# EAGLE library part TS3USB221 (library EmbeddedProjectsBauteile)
USB-Hub
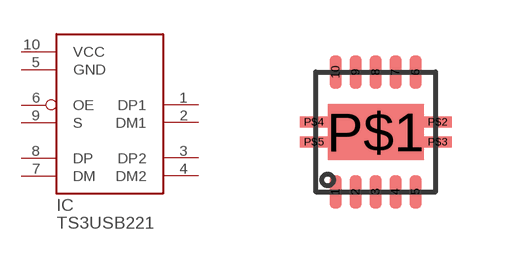
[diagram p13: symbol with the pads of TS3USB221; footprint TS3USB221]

Designator prefix IC

## TS3USB221 (EP: 400184)  [TS3USB221]
1  DP1
2  DM1
3  DP2
4  DM2
5  GND
6  OE
7  DM
8  DP
9  S
10  VCC  pwr

## Footprint TS3USB221 (pad centres in mm)
smd 0.3 x 0.85: 1 -1,-1.5; 2 -0.5,-1.5; 3 0,-1.5; 4 0.5,-1.5; 5 1,-1.5; 6 1,1.5; 7 0.5,1.5; 8 0,1.5; 9 -0.5,1.5; 10 -1,1.5
smd 2.4 x 1.4: P$1 0,0
smd 0.7 x 0.28: P$2 1.55,0.25; P$3 1.55,-0.25; P$4 -1.55,0.25; P$5 -1.55,-0.25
